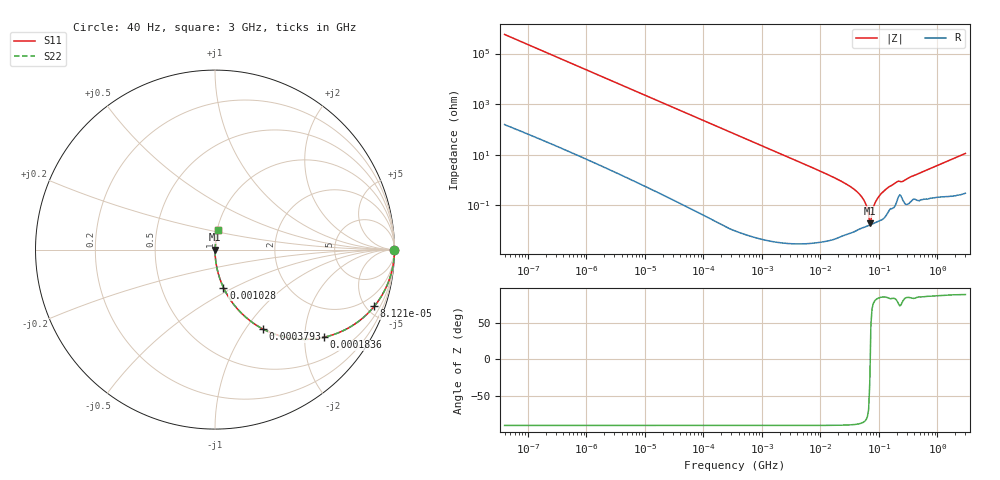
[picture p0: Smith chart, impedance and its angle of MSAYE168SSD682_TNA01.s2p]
! MSAYE168SSD682_TNA01  S-PARAMETER MODEL  ( General Type )
! Model Generated by TAIYO YUDEN Corporation (http://www.ty-top.com)
! Version 2.0
! TAIYO YUDEN Control No. 030711
! Copyright(c) 2003 TAIYO YUDEN CO.,LTD. All Rights Reserved.
! Product Description (link to TY-COMPAS)
! https://ds.yuden.co.jp/TYCOMPAS/or/detail?pn=MSAYE168SSD682KTNA01&u=M
! Products Name : Multilayer Ceramic Capacitors
! Characteristics :
!  Capacitance : 6800 pF , Rated Voltage : 16V
!  Case Size : 1.6 x 0.8 / 0.063 x 0.031 [mm/inch] , Thickness : 0.8 / 0.031 [mm/inch]
!  (Conditions: Temperature = 25 degC , DC Bias Current/Voltage = 0A / 0V)
! External Node Assignments :
!  1  o---| |---o  2
! GND o---------o GND
! Frequency Range : 40Hz  -  3GHz  [ 401 STEP ]
# MHz S RI R 50
! Freq[MHz].  S11 Real  S11 Imag  S21 Real  S21 Imag  S12 Real  S12 Imag  S22 Real  S22 Imag
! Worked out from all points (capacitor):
!   401 points, 40 Hz to 3 GHz, reference 50 ohm
!   read as one part in series: C = 6.98 nF near 44 Hz
!   lowest |Z| = 19.5 mohm at 69.67 MHz (marker M1)
!   series resonance near 70.78 MHz, so ESL is about 720 pH
!   S11 on the Smith chart (normalised r, x): 40 Hz: open; 81.21 kHz: 1.00, -5.61; 183.6 kHz: 1.00, -2.48; 379.3 kHz: 1.00, -1.20; 1.028 MHz: 1.00, -0.44; 3 GHz: 1.01, +0.23
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4e-05  1 -0.000175  7.9e-08 0.000175  7.9e-08 0.000175  1 -0.000175
0.000834  1 -0.00366  1.45e-05 0.00366  1.45e-05 0.00366  1 -0.00366
0.017386  0.9942 -0.0758  0.0058 0.0758  0.0058 0.0758  0.9942 -0.0758
0.081206  0.8873 -0.3161  0.1127 0.3161  0.1127 0.3161  0.8873 -0.3161
0.183638  0.6064 -0.4885  0.3936 0.4885  0.3936 0.4885  0.6064 -0.4885
0.362475  0.2834 -0.4506  0.7166 0.4506  0.7166 0.4506  0.2834 -0.4506
0.379285  0.2654 -0.4415  0.7346 0.4415  0.7346 0.4415  0.2654 -0.4415
1.02824  0.0469 -0.2112  0.9531 0.2112  0.9531 0.2112  0.0469 -0.2112
7.222098  0.00101 -0.0312  0.999 0.0312  0.999 0.0312  0.00101 -0.0312
22.43131  0.000141 -0.00911  0.9999 0.00911  0.9999 0.00911  0.000141 -0.00911
40.43842  0.000112 -0.00376  0.9999 0.00376  0.9999 0.00376  0.000112 -0.00376
55.54024  0.000138 -0.00157  0.9999 0.00157  0.9999 0.00157  0.000138 -0.00157
60.81113  0.000146 -0.000977  0.9999 0.000977  0.9999 0.000977  0.000146 -0.000977
66.58224  0.000158 -0.000397  0.9998 0.000397  0.9998 0.000397  0.000158 -0.000397
69.67004  0.000165 -0.000103  0.9998 0.000103  0.9998 0.000103  0.000165 -0.000103
76.28187  0.000183 0.000484  0.9998 -0.000484  0.9998 -0.000484  0.000183 0.000484
83.52119  0.000203 0.00107  0.9998 -0.00107  0.9998 -0.00107  0.000203 0.00107
95.68847  0.000236 0.00196  0.9998 -0.00196  0.9998 -0.00196  0.000236 0.00196
150.5692  0.000681 0.00548  0.9993 -0.00548  0.9993 -0.00548  0.000681 0.00548
206.7996  0.00176 0.00855  0.9982 -0.00855  0.9982 -0.00855  0.00176 0.00855
259.4108  0.0016 0.00891  0.9984 -0.00891  0.9984 -0.00891  0.0016 0.00891
3000  0.0155 0.111  0.9845 -0.111  0.9845 -0.111  0.0155 0.111
